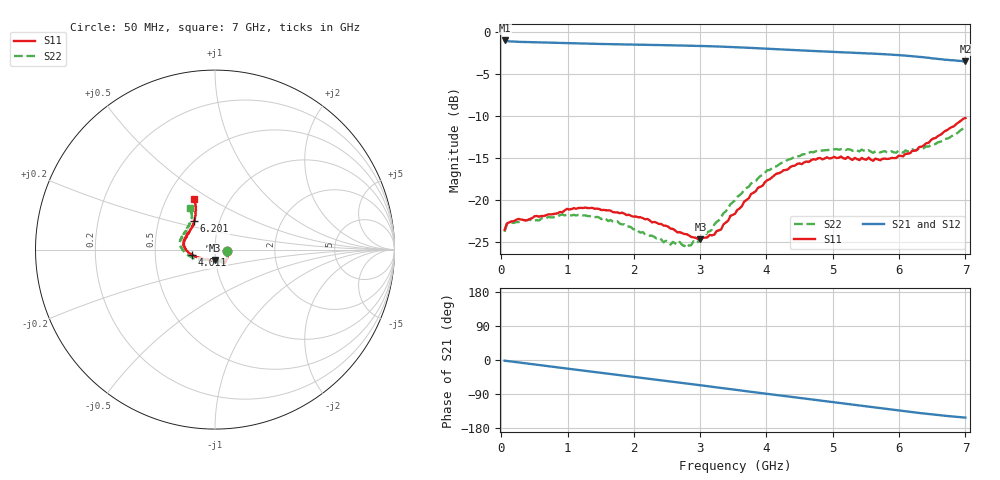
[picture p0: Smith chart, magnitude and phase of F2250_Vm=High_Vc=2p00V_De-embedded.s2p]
! Integrated Device Technology
! Corporate Headquarters
! 6024 Silver Creek Valley Road
! San Jose, CA 95138  USA
! Phone:  1-408-284-8200
! Toll Free:  1-800-223-1366
! Webpage:  http://www.idt.com/
! Timing and RF Division
! 515 Groton Road, Suite 102
! Westford, MA 01886-6024
! Device:  F2250
! Description: Voltage Variable RF Attenuator
! Frequency:  50.0 -  6000.00 MHz
! Package:  3x3 mm Thin QFN Plastic Package: 16 pin
! Ports:  2 RF, 3 DC
!  Pin  1  = GND
!  Pin  2  = NC
!  Pin  3  = RF1  = Port 1
!  Pin  4  = NC
!  Pin  5  = GND
!  Pin  6  = GND
!  Pin  7  = GND
!  Pin  8  = GND
!  Pin  9  = NC
!  Pin 10  = RF2  = Port 2
!  Pin 11  = NC
!  Pin 12  = GND
!  Pin 13  = GND
!  Pin 14  = VCNTRL
!  Pin 15  = VDD
!  Pin 16  = VMODE
! Vcntrl:  2.000 Volts
! Vmode:  +3.300 Volts
! Vdd:  +3.30  Volts
! Current:  1.321 mA
! Data:  The device was measured on a the F2250 evaluation board which has
!  individual transmission lines to the RF pins.  Data was collected
!  using a calibrated network analyzer.  The evaluation board was
!  de-embedded using a TRL calibration technique.
!  The reference plane is the edge of the package pin.
! Misc:  SN 10
!  Action Tracker AT0258
! Date Measured:  2014-11-26
! Date:  2015-10-15  MJV
! Note:
!  Integrated Device Technology supplies this data as a sample of measured
!  data at the package pin for this product.  Your particular data for this
!  product may vary.
!  Data was taken at 25 degrees C.
!  Integrated Device Technology reserves the right to change this data at anytime.
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# GHz S dB R 50
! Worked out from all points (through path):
!   201 points, 50 MHz to 7 GHz, reference 50 ohm
!   highest |S21| = -1.03 dB at 50 MHz (marker M1); lowest = -3.5 dB at 7 GHz (marker M2)
!   group delay of S21, straight-line fit = 61.1 ps
!   lowest |S11| = -24.7 dB at 3.004 GHz (marker M3), VSWR 1.12, Z = 49.4 - j5.79 ohm
!   |S11| at or under -10 dB: start of sweep to end of sweep
!   |S22| runs from -25.5 to -11.4 dB; largest |S21 - S12| = 0.0019
!   S11 on the Smith chart (normalised r, x): 50 MHz: 1.14, -0.02; 4.011 GHz: 0.77, -0.05; 6.201 GHz: 0.75, +0.25; 7 GHz: 0.68, +0.43
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0.05  -23.53 -8.5  -1.03 -1.8  -1.03 -1.8  -23.75 -9.2
0.08475  -22.76 -7.8  -1.11 -2.5  -1.11 -2.5  -22.87 -8.2
0.1195  -22.64 -8.4  -1.14 -3.3  -1.14 -3.2  -22.69 -7.9
0.91875  -21.44 -43.6  -1.33 -21.1  -1.33 -21.1  -21.69 -47.1
1.2315  -20.93 -51.4  -1.40 -27.9  -1.40 -27.9  -21.80 -57.4
1.75275  -21.46 -58.3  -1.49 -39.1  -1.49 -39.1  -22.52 -65.5
2.37825  -22.83 -59.1  -1.58 -52.7  -1.58 -52.7  -24.51 -69.8
2.552  -23.38 -63.3  -1.60 -56.6  -1.60 -56.6  -25.28 -76.4
2.691  -23.80 -69.7  -1.63 -59.7  -1.63 -59.7  -24.96 -83.2
2.7605  -24.02 -71.6  -1.64 -61.2  -1.64 -61.3  -25.47 -87.3
3.00375  -24.67 -92.4  -1.69 -66.7  -1.69 -66.7  -24.50 -108.5
3.21225  -24.10 -113.9  -1.73 -71.4  -1.73 -71.4  -22.91 -126.6
3.525  -21.63 -142.1  -1.83 -78.5  -1.83 -78.5  -20.02 -145.4
3.76825  -19.26 -156.9  -1.92 -84.0  -1.92 -84.0  -18.02 -156.8
4.0115  -17.63 -166.7  -2.02 -89.4  -2.02 -89.4  -16.44 -166.6
4.4285  -15.90 -179.0  -2.18 -98.6  -2.18 -98.6  -14.80 -179.5
4.7065  -15.13 173.6  -2.28 -104.8  -2.28 -104.8  -14.32 174.5
5.054  -14.99 165.3  -2.41 -112.4  -2.40 -112.5  -13.93 167.2
5.85325  -15.08 138.8  -2.70 -129.9  -2.70 -130.0  -14.33 148.1
6.20075  -14.12 126.6  -2.91 -137.6  -2.91 -137.7  -13.95 138.9
6.54825  -12.62 118.0  -3.18 -144.6  -3.18 -144.8  -13.33 127.5
7  -10.24 112.7  -3.51 -152.0  -3.52 -152.1  -11.38 121.2
